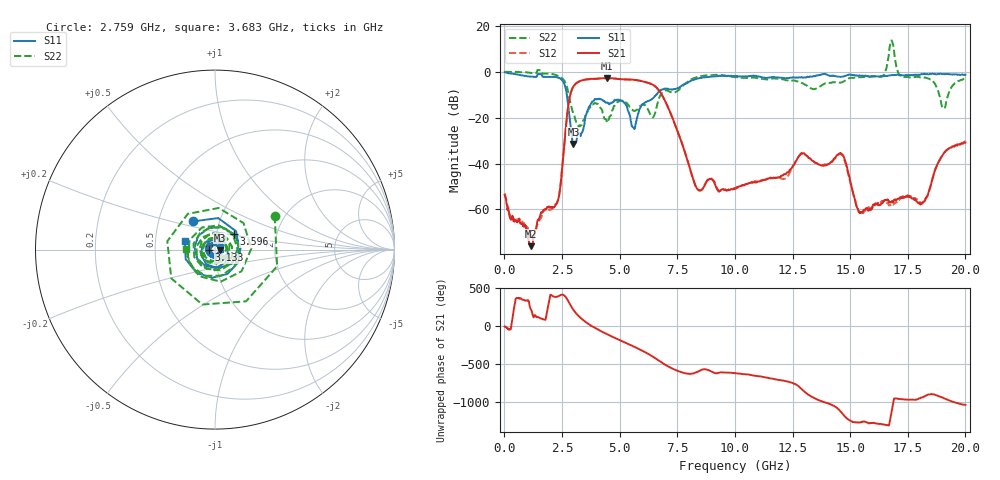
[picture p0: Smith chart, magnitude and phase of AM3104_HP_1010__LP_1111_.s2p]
!Created with skrf (http://scikit-rf.org).
# Hz S RI R 50.0
!freq ReS11 ImS11 ReS21 ImS21 ReS12 ImS12 ReS22 ImS22
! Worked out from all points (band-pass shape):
!   1601 points, 10 MHz to 20 GHz, reference 50 ohm
!   highest |S21| = -2.76 dB at 4.458 GHz (marker M1); lowest = -76.0 dB at 1.134 GHz (marker M2)
!   |S21| within 3 dB of the highest: 3.046 GHz to 6.457 GHz (3.411 GHz wide, 71.8 % of centre)
!   lowest |S11| = -31.5 dB at 2.996 GHz (marker M3), VSWR 1.05, Z = 52.7 - j0.174 ohm
!   |S11| at or under -10 dB: 2.71 GHz to 6.594 GHz (3.885 GHz wide, 83.5 % of centre)
!   |S22| runs from -24.2 to 13.6 dB; largest |S21 - S12| = 0.083
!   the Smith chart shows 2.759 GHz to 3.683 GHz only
!   S11 on the Smith chart (normalised r, x): 2.759 GHz: 0.75, +0.25; 3.133 GHz: 0.94, -0.01; 3.596 GHz: 1.22, +0.21; 3.683 GHz: 0.71, +0.07
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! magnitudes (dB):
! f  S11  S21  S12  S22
! 10 MHz  -0.2  -53.6  -53.1  -0.1
! 1.134 GHz  -2.1  -76.0  -71.3  -0.5
! 2.321 GHz  -2.5  -56.1  -56.1  -1.8
! 2.759 GHz  -14.0  -15.9  -15.9  -8.4
! 2.996 GHz  -31.5  -6.4  -6.4  -18.3
! 3.133 GHz  -29.9  -4.9  -4.9  -22.1
! 3.346 GHz  -26.7  -3.8  -3.9  -23.2
! 3.596 GHz  -17.2  -3.3  -3.4  -17.7
! 3.683 GHz  -15.2  -3.2  -3.3  -15.7
! 4.458 GHz  -13.4  -2.8  -2.8  -22.2
! 5.607 GHz  -24.5  -3.5  -3.5  -17.0
! 6.682 GHz  -8.9  -7.8  -7.8  -12.4
! 8.368 GHz  -3.0  -51.1  -51.0  -2.2
! 10.01 GHz  -2.0  -50.9  -50.7  -2.4
! 13.34 GHz  -2.2  -38.7  -38.6  -7.5
! 14.65 GHz  -2.2  -36.0  -36.4  -4.6
! 15.45 GHz  -1.8  -61.4  -61.6  -2.4
! 16.4 GHz  -1.9  -57.3  -56.4  -1.9
! 16.68 GHz  -1.7  -56.6  -57.9  7.3
! 18.15 GHz  -1.1  -56.8  -57.0  -2.4
! 19.05 GHz  -1.0  -35.7  -35.6  -15.9
! 20 GHz  -1.3  -30.8  -30.4  -3.0
